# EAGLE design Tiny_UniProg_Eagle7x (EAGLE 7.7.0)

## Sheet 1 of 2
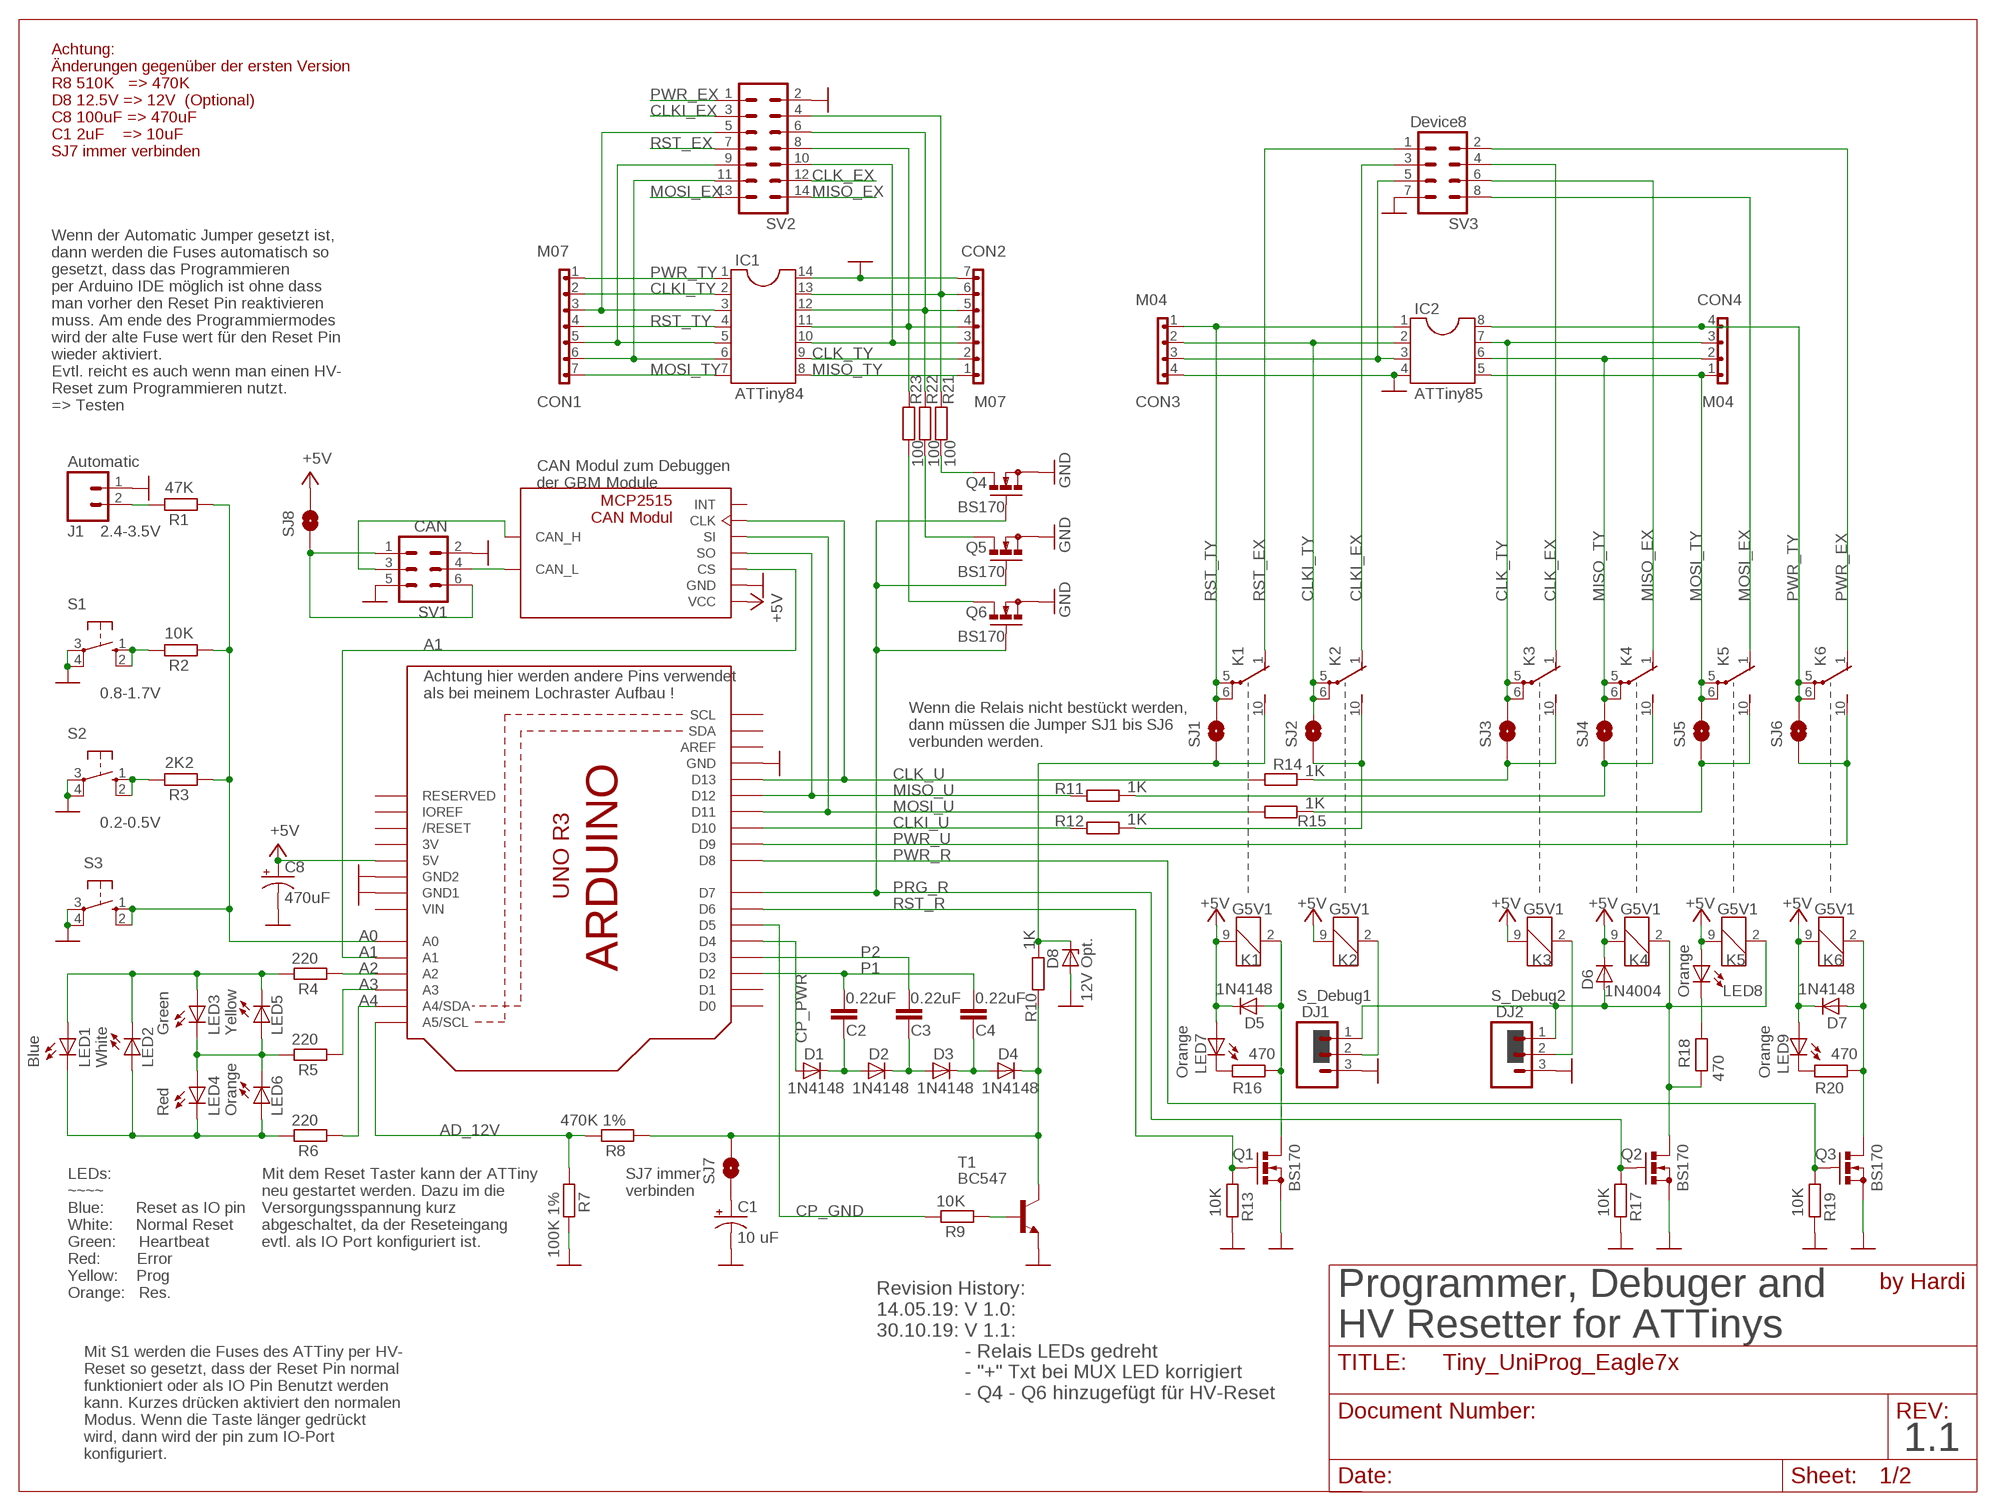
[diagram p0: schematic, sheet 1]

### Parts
C1  10 uF  100UF-25V-20%(PTH)D5MM  [CPOL-RADIAL-10UF-63V]
C2  0.22uF  C-EU050-024X044  [C050-024X044]
C3  0.22uF  C-EU050-024X044  [C050-024X044]
C4  0.22uF  C-EU050-024X044  [C050-024X044]
C8  470uF  SPARKFUN-CAPACITORS_100UF-25V-20%(PTH)  [SPARKFUN-CAPACITORS_CPOL-RADIAL-100UF-25V]
CAN1  MCP2515_CAN_MODUL  [MCP2515_CAN_MODUL]
CON1  M07  [1X07]
CON2  M07  [1X07]
CON3  M04  [1X04]
CON4  M04  [1X04]
D1  1N4148  1N4148DO35-2  [DO35-2]
D2  1N4148  1N4148DO35-2  [DO35-2]
D3  1N4148  1N4148DO35-2  [DO35-2]
D4  1N4148  1N4148DO35-2  [DO35-2]
D5  1N4148  1N4148DO35-2  [DO35-2]
D6  1N4004  1N4004DO35-2  [DO35-2]
D7  1N4148  1N4148DO35-2  [DO35-2]
D8  12V Opt.  ZENER-DIODEZD-2.5  [ZDIO-2.5]
DJ1  S_Debug1  M03PTH  [1X03]
DJ2  S_Debug2  M03PTH  [1X03]
IC1  ATTiny84  DIL14  [DIL14]
IC2  ATTiny85  DIL8  [DIL08]
J1  Automatic  M02PTH  [1X02]
K1  G5V1  [G5V1]
K2  G5V1  [G5V1]
K3  G5V1  [G5V1]
K4  G5V1  [G5V1]
K5  G5V1  [G5V1]
K6  G5V1  [G5V1]
LED1  Blue  LED3MM  [LED3MM]
LED2  White  LED3MM  [LED3MM]
LED3  Green  LED3MM  [LED3MM]
LED4  Red  LED3MM  [LED3MM]
LED5  Yellow  LED3MM  [LED3MM]
LED6  Orange  LED3MM  [LED3MM]
LED7  Orange  LED3MM  [LED3MM]
LED8  Orange  LED3MM  [LED3MM]
LED9  Orange  LED3MM  [LED3MM]
Q1  BS170  [SOT54E]
Q2  BS170  [SOT54E]
Q3  BS170  [SOT54E]
Q4  BS170  [SOT54E]
Q5  BS170  [SOT54E]
Q6  BS170  [SOT54E]
R1  47K  R0204/7  [0204/7]
R2  10K  R0204/7  [0204/7]
R3  2K2  R0204/2V  [0204/2V]
R4  220  R0204/2V  [0204/2V]
R5  220  R0204/2V  [0204/2V]
R6  220  R0204/2V  [0204/2V]
R7  100K 1%  R0204/2V  [0204/2V]
R8  470K 1%  R0204/7  [0204/7]
R9  10K  R0204/2V  [0204/2V]
R10  1K  R0204/2V  [0204/2V]
R11  1K  R0204/2V  [0204/2V]
R12  1K  R0204/2V  [0204/2V]
R13  10K  R0204/2V  [0204/2V]
R14  1K  R0204/2V  [0204/2V]
R15  1K  R0204/2V  [0204/2V]
R16  470  R0204/2V  [0204/2V]
R17  10K  R0204/2V  [0204/2V]
R18  470  R0204/2V  [0204/2V]
R19  10K  R0204/2V  [0204/2V]
R20  470  R0204/2V  [0204/2V]
R21  100  R0204/2V  [0204/2V]
R22  100  R0204/2V  [0204/2V]
R23  100  R0204/2V  [0204/2V]
S1  10-XX  [B3F-10XX]
S2  10-XX  [B3F-10XX]
S3  10-XX  [B3F-10XX]
SJ1  SOLDERJUMPERNO  [SJ_2S-NO]
SJ2  SOLDERJUMPERNO  [SJ_2S-NO]
SJ3  SOLDERJUMPERNO  [SJ_2S-NO]
SJ4  SOLDERJUMPERNO  [SJ_2S-NO]
SJ5  SOLDERJUMPERNO  [SJ_2S-NO]
SJ6  SOLDERJUMPERNO  [SJ_2S-NO]
SJ7  SOLDERJUMPERNO  [SJ_2S-NO]
SJ8  SOLDERJUMPERNO  [SJ_2S-NO]
SV1  CAN  ML6  [ML6]
SV2  ML14  [ML14]
SV3  Device8  CON-HARTING-ML_ML08  [CON-HARTING-ML_ML08]
T1  BC547  [TO92]
U1  ARDUINOR3-DIMENSION  [ARDUINOR3]

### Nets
+5V: C8.1(+) CAN1.1(VCC) D5.C D6.C D7.C K1.9 K2.9 K3.9 K4.9 K5.9 K6.9 LED7.A LED8.A LED9.A SJ8.2 U1.5V
A0: R1.1 R2.1 R3.1 S3.1(S) S3.2(S1) U1.A0
A1: CAN1.3(CS) U1.A1
A2: R4.1 U1.A2
A3: R5.1 U1.A3
A4: R6.1 U1.A4(A4/SDA)
AD_12V: R7.1 R8.2 U1.A5(A5/SCL)
CLK_EX: K3.1(2:O) SV2.12 SV3.4
CLK_TY: CON2.2 CON4.3 IC1.9 IC2.7 K3.5(2:P) K3.6(2:P) SJ3.2
CLK_U: CAN1.6(CLK) R14.1 U1.D13
CLKI_EX: K2.1(2:O) SV2.3 SV3.3
CLKI_TY: CON1.2 CON3.2 IC1.2 IC2.2 K2.5(2:P) K2.6(2:P) SJ2.2
CLKI_U: R12.1 U1.D10
CP_GND: R9.2 U1.D5
CP_PWR: D1.A U1.D4
GND: C1.2(-) C8.2(-) CAN1.2(GND) CON2.7 CON3.4 D8.A DJ1.3 DJ2.3 IC1.14 IC2.4 J1.1 Q1.S Q2.S Q3.S Q4.S Q5.S Q6.S R7.2 R13.2 R17.2 R19.2 S1.3(P) S1.4(P1) S2.3(P) S2.4(P1) S3.3(P) S3.4(P1) SV1.2 SV1.5 SV2.2 SV3.7 T1.1(E) U1.GND U1.GND1 U1.GND2
MISO_EX: K4.1(2:O) SV2.14 SV3.6
MISO_TY: CON2.1 CON4.2 IC1.8 IC2.6 K4.5(2:P) K4.6(2:P) SJ4.2
MISO_U: CAN1.4(SO) R11.1 U1.D12
MOSI_EX: K5.1(2:O) SV2.13 SV3.8
MOSI_TY: CON1.7 CON4.1 IC1.7 IC2.5 K5.5(2:P) K5.6(2:P) SJ5.2
MOSI_U: CAN1.5(SI) R15.1 U1.D11
N$1: C2.2 D1.C D2.A
N$2: C3.2 D2.C D3.A
N$3: C4.2 D3.C D4.A
N$6: CON2.3 IC1.10 SV2.10
N$7: R9.1 T1.2(B)
N$8: CAN1.8(CAN_L) SV1.4
N$9: D4.C R8.1 R10.2 SJ7.2 T1.3(C)
N$10: CAN1.9(CAN_H) SV1.3
N$11: CON2.4 IC1.11 R23.2 SV2.8
N$12: CON2.5 IC1.12 R22.2 SV2.6
N$13: K5.10(2:S) R15.2 SJ5.1
N$14: CON2.6 IC1.13 R21.2 SV2.4
N$15: K4.10(2:S) R11.2 SJ4.1
N$17: K3.10(2:S) R14.2 SJ3.1
N$19: DJ1.2 K2.2
N$20: D5.A K1.2 Q1.D R16.2
N$21: DJ2.2 K3.2
N$22: D8.C K1.10(2:S) R10.1 SJ1.1
N$23: CON1.6 IC1.6 SV2.11
N$24: K2.10(2:S) R12.2 SJ2.1
N$25: D7.A K6.2 Q3.D R20.2
N$26: D6.A DJ1.1 DJ2.1 K4.2 K5.2 Q2.D R18.2
N$27: CON1.5 IC1.5 SV2.9
N$28: J1.2 R1.2
N$30: CON1.3 IC1.3 SV2.5
N$33: R3.2 S2.1(S) S2.2(S1)
N$34: LED1.A LED2.K(C) LED3.A LED5.K(C) R4.2
N$36: LED7.K(C) R16.1
N$37: LED8.K(C) R18.1
N$38: LED9.K(C) R20.1
N$39: C1.1(+) SJ7.1
N$42: LED3.K(C) LED4.A LED5.A LED6.K(C) R5.2
N$44: LED1.K(C) LED2.A LED4.K(C) LED6.A R6.2
N$45: SJ8.1 SV1.1 SV1.6
N$48: CON3.3 IC2.3 SV3.5
N$67: R2.2 S1.1(S) S1.2(S1)
N$108: Q4.D R21.1
N$109: Q5.D R22.1
N$110: Q6.D R23.1
P1: C2.1 C4.1 U1.D2
P2: C3.1 U1.D3
PRG_R: Q2.G Q4.G Q5.G Q6.G R17.1 U1.D7
PWR_EX: K6.1(2:O) SV2.1 SV3.2
PWR_R: Q3.G R19.1 U1.D8
PWR_TY: CON1.1 CON4.4 IC1.1 IC2.8 K6.5(2:P) K6.6(2:P) SJ6.2
PWR_U: K6.10(2:S) SJ6.1 U1.D9
RST_EX: K1.1(2:O) SV2.7 SV3.1
RST_R: Q1.G R13.1 U1.D6
RST_TY: CON1.4 CON3.1 IC1.4 IC2.1 K1.5(2:P) K1.6(2:P) SJ1.2
Unconnected: CAN1.7(INT) U1.AREF U1.D0 U1.D1 U1.IOREF U1.RESERVED U1.RESET(/RESET) U1.SCL U1.SDA

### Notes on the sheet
- Achtung:
  Änderungen gegenüber der ersten Version
  R8 510K   => 470K
  D8 12.5V => 12V  (Optional)
  C8 100uF => 470uF
  C1 2uF    => 10uF
  SJ7 immer verbinden
- Wenn der Automatic Jumper gesetzt ist,
  dann werden die Fuses automatisch so
  gesetzt, dass das Programmieren
  per Arduino IDE möglich ist ohne dass
  man vorher den Reset Pin reaktivieren
  muss. Am ende des Programmiermodes
  wird der alte Fuse wert für den Reset Pin
  wieder aktiviert.
  Evtl. reicht es auch wenn man einen HV-
  Reset zum Programmieren nutzt.
  => Testen
- CAN Modul zum Debuggen 
  der GBM Module
- 2.4-3.5V
- 0.8-1.7V
- Achtung hier werden andere Pins verwendet
  als bei meinem Lochraster Aufbau !
- Wenn die Relais nicht bestückt werden,
  dann müssen die Jumper SJ1 bis SJ6
  verbunden werden.
- 0.2-0.5V
- LEDs:
  ~~~~
  Blue:       Reset as IO pin
  White:     Normal Reset
  Green:     Heartbeat
  Red:        Error
  Yellow:    Prog
  Orange:   Res.
- Mit dem Reset Taster kann der ATTiny
  neu gestartet werden. Dazu im die
  Versorgungsspannung kurz
  abgeschaltet, da der Reseteingang
  evtl. als IO Port konfiguriert ist.
- SJ7 immer
  verbinden
- Revision History:
  14.05.19: V 1.0: 
  30.10.19: V 1.1: 
                  - Relais LEDs gedreht 
                  - "+" Txt bei MUX LED korrigiert
                  - Q4 - Q6 hinzugefügt für HV-Reset
- by Hardi
- Programmer, Debuger and 
  HV Resetter for ATTinys
- Mit S1 werden die Fuses des ATTiny per HV-
  Reset so gesetzt, dass der Reset Pin normal
  funktioniert oder als IO Pin Benutzt werden
  kann. Kurzes drücken aktiviert den normalen
  Modus. Wenn die Taste länger gedrückt
  wird, dann wird der pin zum IO-Port 
  konfiguriert.
- 1.1

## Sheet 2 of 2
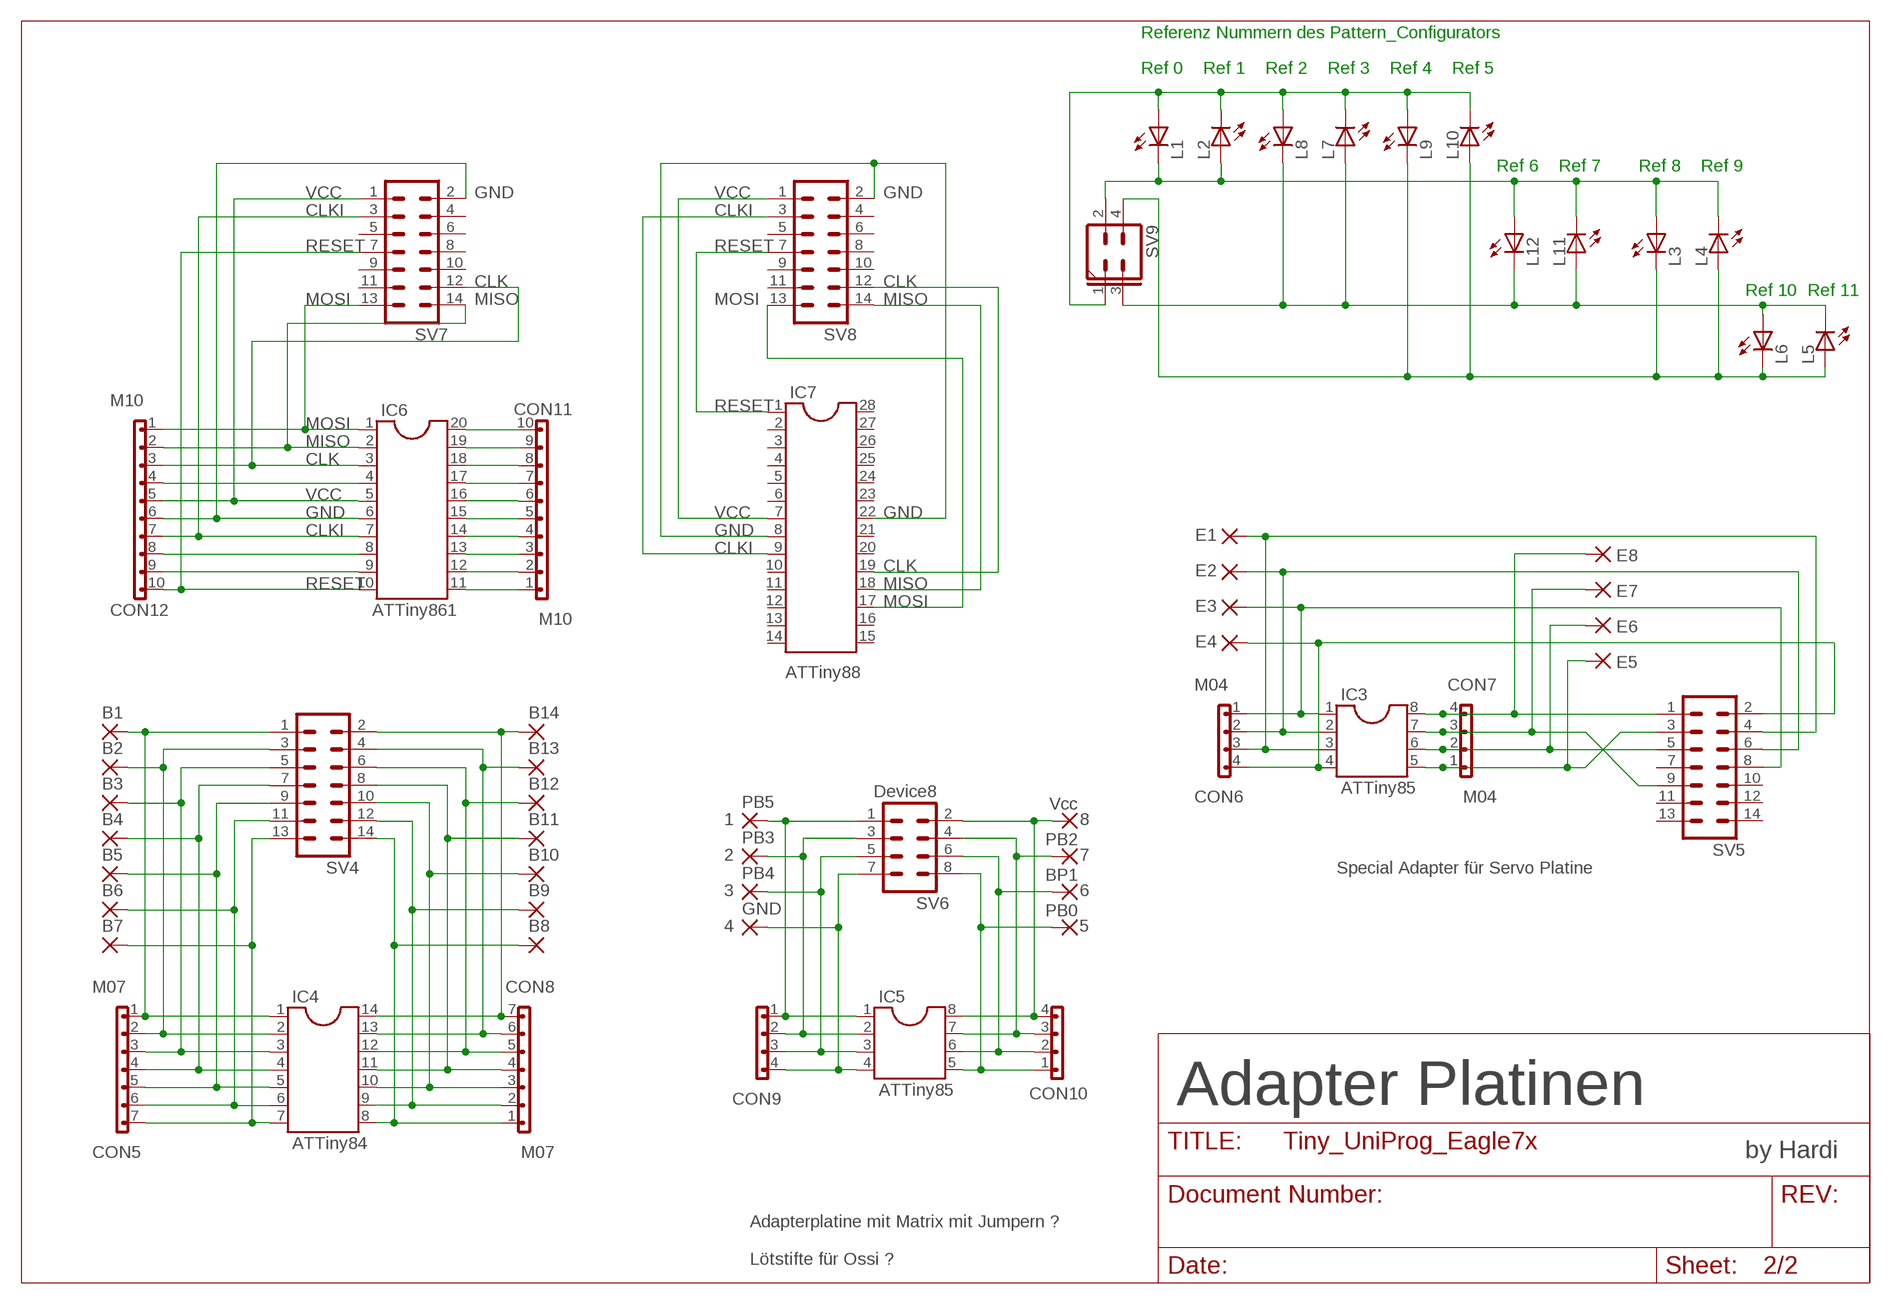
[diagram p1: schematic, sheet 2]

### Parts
1  PB5  2,54/1,0  [2,54/1,0]
2  PB3  2,54/1,0  [2,54/1,0]
3  PB4  2,54/1,0  [2,54/1,0]
4  GND  2,54/1,0  [2,54/1,0]
5  PB0  2,54/1,0  [2,54/1,0]
6  BP1  2,54/1,0  [2,54/1,0]
7  PB2  2,54/1,0  [2,54/1,0]
8  Vcc  2,54/1,0  [2,54/1,0]
B1  2,54/1,0  [2,54/1,0]
B2  2,54/1,0  [2,54/1,0]
B3  2,54/1,0  [2,54/1,0]
B4  2,54/1,0  [2,54/1,0]
B5  2,54/1,0  [2,54/1,0]
B6  2,54/1,0  [2,54/1,0]
B7  2,54/1,0  [2,54/1,0]
B8  2,54/1,0  [2,54/1,0]
B9  2,54/1,0  [2,54/1,0]
B10  2,54/1,0  [2,54/1,0]
B11  2,54/1,0  [2,54/1,0]
B12  2,54/1,0  [2,54/1,0]
B13  2,54/1,0  [2,54/1,0]
B14  2,54/1,0  [2,54/1,0]
CON5  M07  [1X07]
CON6  M04  [1X04]
CON7  M04  [1X04]
CON8  M07  [1X07]
CON9  M04  [1X04]
CON10  M04  [1X04]
CON11  M10  [1X10]
CON12  M10  [1X10]
E1  2,54/1,0  [2,54/1,0]
E2  2,54/1,0  [2,54/1,0]
E3  2,54/1,0  [2,54/1,0]
E4  2,54/1,0  [2,54/1,0]
E5  2,54/1,0  [2,54/1,0]
E6  2,54/1,0  [2,54/1,0]
E7  2,54/1,0  [2,54/1,0]
E8  2,54/1,0  [2,54/1,0]
IC3  ATTiny85  DIL8  [DIL08]
IC4  ATTiny84  DIL14  [DIL14]
IC5  ATTiny85  DIL8  [DIL08]
IC6  ATTiny861  DIL20  [DIL20]
IC7  DIL28-3  [DIL28-3]
L1  LED3MM  [LED3MM]
L2  LED3MM  [LED3MM]
L3  LED3MM  [LED3MM]
L4  LED3MM  [LED3MM]
L5  LED3MM  [LED3MM]
L6  LED3MM  [LED3MM]
L7  LED3MM  [LED3MM]
L8  LED3MM  [LED3MM]
L9  LED3MM  [LED3MM]
L10  LED3MM  [LED3MM]
L11  LED3MM  [LED3MM]
L12  LED3MM  [LED3MM]
SV4  ML14  [ML14]
SV5  ML14  [ML14]
SV6  Device8  CON-HARTING-ML_ML08  [CON-HARTING-ML_ML08]
SV7  ML14  [ML14]
SV8  ML14  [ML14]
SV9  MA02-2MUX-SIGNAL  [MUX-SIGNAL]

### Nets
N$4: 4.1(P) CON9.4 IC5.4 SV6.7
N$5: 3.1(P) CON9.3 IC5.3 SV6.5
N$16: 2.1(P) CON9.2 IC5.2 SV6.3
N$18: 1.1(P) CON9.1 IC5.1 SV6.1
N$29: 5.1(P) CON10.1 IC5.5 SV6.8
N$31: 6.1(P) CON10.2 IC5.6 SV6.6
N$32: 7.1(P) CON10.3 IC5.7 SV6.4
N$35: B8.1(P) CON8.1 IC4.8 SV4.14
N$40: B9.1(P) CON8.2 IC4.9 SV4.12
N$41: B10.1(P) CON8.3 IC4.10 SV4.10
N$43: B11.1(P) CON8.4 IC4.11 SV4.8
N$46: B12.1(P) CON8.5 IC4.12 SV4.6
N$47: B13.1(P) CON8.6 IC4.13 SV4.4
N$49: B14.1(P) CON8.7 IC4.14 SV4.2
N$50: B7.1(P) CON5.7 IC4.7 SV4.13
N$51: B6.1(P) CON5.6 IC4.6 SV4.11
N$52: B5.1(P) CON5.5 IC4.5 SV4.9
N$53: B4.1(P) CON5.4 IC4.4 SV4.7
N$54: B3.1(P) CON5.3 IC4.3 SV4.5
N$55: B2.1(P) CON5.2 IC4.2 SV4.3
N$56: B1.1(P) CON5.1 IC4.1 SV4.1
N$57: 8.1(P) CON10.4 IC5.8 SV6.2
N$58: CON7.4 E8.1(P) IC3.8 SV5.1
N$59: CON6.4 E4.1(P) IC3.4 SV5.2
N$60: CON7.3 E7.1(P) IC3.7 SV5.9
N$61: CON7.2 E6.1(P) IC3.6 SV5.5
N$62: CON7.1 E5.1(P) IC3.5 SV5.3
N$63: CON6.1 E3.1(P) IC3.1 SV5.8
N$64: CON6.2 E2.1(P) IC3.2 SV5.6
N$65: CON6.3 E1.1(P) IC3.3 SV5.4
N$66: CON12.10 IC6.10 SV7.7
N$68: CON12.7 IC6.7 SV7.3
N$69: CON12.6 IC6.6 SV7.2
N$70: CON12.5 IC6.5 SV7.1
N$71: CON12.3 IC6.3 SV7.12
N$72: CON12.2 IC6.2 SV7.14
N$73: CON12.1 IC6.1 SV7.13
N$74: CON12.4 IC6.4
N$75: CON12.8 IC6.8
N$76: CON12.9 IC6.9
N$77: CON11.1 IC6.11
N$78: CON11.2 IC6.12
N$79: CON11.3 IC6.13
N$80: CON11.4 IC6.14
N$81: CON11.5 IC6.15
N$82: CON11.6 IC6.16
N$83: CON11.7 IC6.17
N$84: CON11.8 IC6.18
N$85: CON11.9 IC6.19
N$86: CON11.10 IC6.20
N$87: IC7.9 SV8.3
N$88: IC7.8 IC7.22 SV8.2
N$89: IC7.7 SV8.1
N$90: IC7.1 SV8.7
N$91: IC7.17 SV8.13
N$92: IC7.18 SV8.14
N$93: L1.K(C) L2.A L3.A L4.K(C) L11.K(C) L12.A SV9.2
N$94: IC7.19 SV8.12
N$95: L1.A L2.K(C) L7.K(C) L8.A L9.A L10.K(C) SV9.1
N$97: L3.K(C) L4.A L5.A L6.K(C) L9.K(C) L10.A SV9.4
N$98: L5.K(C) L6.A L7.A L8.K(C) L11.A L12.K(C) SV9.3
Unconnected: IC7.2 IC7.3 IC7.4 IC7.5 IC7.6 IC7.10 IC7.11 IC7.12 IC7.13 IC7.14 IC7.15 IC7.16 IC7.20 IC7.21 IC7.23 IC7.24 IC7.25 IC7.26 IC7.27 IC7.28 SV5.7 SV5.10 SV5.11 SV5.12 SV5.13 SV5.14 SV7.4 SV7.5 SV7.6 SV7.8 SV7.9 SV7.10 SV7.11 SV8.4 SV8.5 SV8.6 SV8.8 SV8.9 SV8.10 SV8.11

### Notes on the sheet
- Referenz Nummern des Pattern_Configurators
- Ref 0 | Ref 1 | Ref 2 | Ref 3 | Ref 4 | Ref 5
- Ref 6 | Ref 7 | Ref 8 | Ref 9
- VCC | GND | VCC | GND
- CLKI | CLKI
- RESET | RESET
- CLK | CLK
- Ref 10 | Ref 11
- MOSI | MISO | MOSI | MISO
- RESET
- MOSI
- MISO
- CLK
- VCC
- GND | VCC | GND
- CLKI | GND
- CLKI
- CLK
- RESET | MISO
- MOSI
- ATTiny88
- Special Adapter für Servo Platine
- Adapter Platinen
- by Hardi
- Adapterplatine mit Matrix mit Jumpern ?
  
  Lötstifte für Ossi ?

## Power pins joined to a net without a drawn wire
3V: U1.3V
VIN: U1.VIN

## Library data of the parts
1-8 B1-B14 E1-E8 = wirepad:2,54/1,0: THROUGH-HOLE PAD
C1 = SparkFun-Capacitors:100UF-25V-20%(PTH): CAP-08439
C2-C4 = rcl:C-EU: CAPACITOR, European symbol; SPICEPREFIX: C
C8 = Sound_MP3-TF-16P_and_WS2811:SPARKFUN-CAPACITORS_100UF-25V-20%(PTH): CAP-08439; PROD_ID: CAP-08439
CAN1 = Arduino_fuer_LEDs_DCC_2_All:MCP2515_CAN_MODUL: MCP2515 CAN Modul
CON1 CON2 CON5 CON8 = Connectors_Inline3_7:M07
CON3 CON4 CON6 CON7 CON9 CON10 = Connectors_Inline3_7:M04
CON11 CON12 = Connectors_Inline3_7:M10
D1-D5 D7 = diode:1N4148: DIODE
D6 = diode:1N4004: DIODE
D8 = diode@1:ZENER-DIODE: Z-Diode
DJ1 DJ2 = SparkFun-Connectors:M03: Header 3 Standard 3-pin 0.1" header. Use with straight break away headers (SKU : PRT-00116), right angle break away headers (PRT-00553), swiss pins (PRT-00743), machine pins (PRT-00117), and female headers (PRT-00115). Molex polarized connector foot print use with SKU : PRT-08232 with associated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
IC1 IC4 = ic-package:DIL14: Dual In Line / Socket
IC2 IC3 IC5 = ic-package:DIL8: Dual In Line / Socket
IC6 = ic-package@1:DIL20: Dual In Line / Socket
IC7 = ic-package@1:DIL28: Dual In Line
J1 = SparkFun-Connectors:M02: Standard 2-pin 0.1" header. Use with
K1-K6 = relay:G5V1: RELAY 1 x switch, 0.5 A/125 V AC, 1 A/24 V DC , Omron; MPN: G5V-1-DC24; OC_FARNELL: 9949593; OC_NEWARK: 36M6377
L1-L12 LED1-LED9 = Arduino_fuer_LEDs_DCC_2:LED: LED
Q1-Q6 = transistor-small-signal:BS170: N-CHANNEL MOS FET
R1 R2 R8 = Arduino_fuer_LEDs_DCC_2:R: RESISTOR, European symbol; SPICEMODEL: NONE; SPICEPREFIX: R
R3-R7 R9-R23 = Arduino_fuer_LEDs_DCC_2:R: RESISTOR, European symbol
S1-S3 = switch-omron:10-XX: OMRON SWITCH; MPN: B3F-1000; OC_FARNELL: 176432; OC_NEWARK: 36M3542
SJ1-SJ8 = SparkFun-Retired:SOLDERJUMPER: Solder Jumper
SV1 = Arduino_fuer_LEDs_DCC_2:ML6: HARTING; OC_FARNELL: unknown; OC_NEWARK: unknown
SV2 SV4 SV5 SV7 SV8 = Arduino_fuer_LEDs_DCC_2:ML14: HARTING; OC_FARNELL: unknown; OC_NEWARK: unknown
SV3 SV6 = PushButtonAction_4017_2:CON-HARTING-ML_ML08: Modified by Hardi; OC_FARNELL: unknown; OC_NEWARK: unknown
SV9 = con-lstb:MA02-2: PIN HEADER
T1 = transistor:BC547: NPN TRANSISTOR
U1 = adafruit:ARDUINOR3: This is a new object for the new Arduino R3 - with extra pins that you may want to use (such as IOref, and duplicated A4/A5

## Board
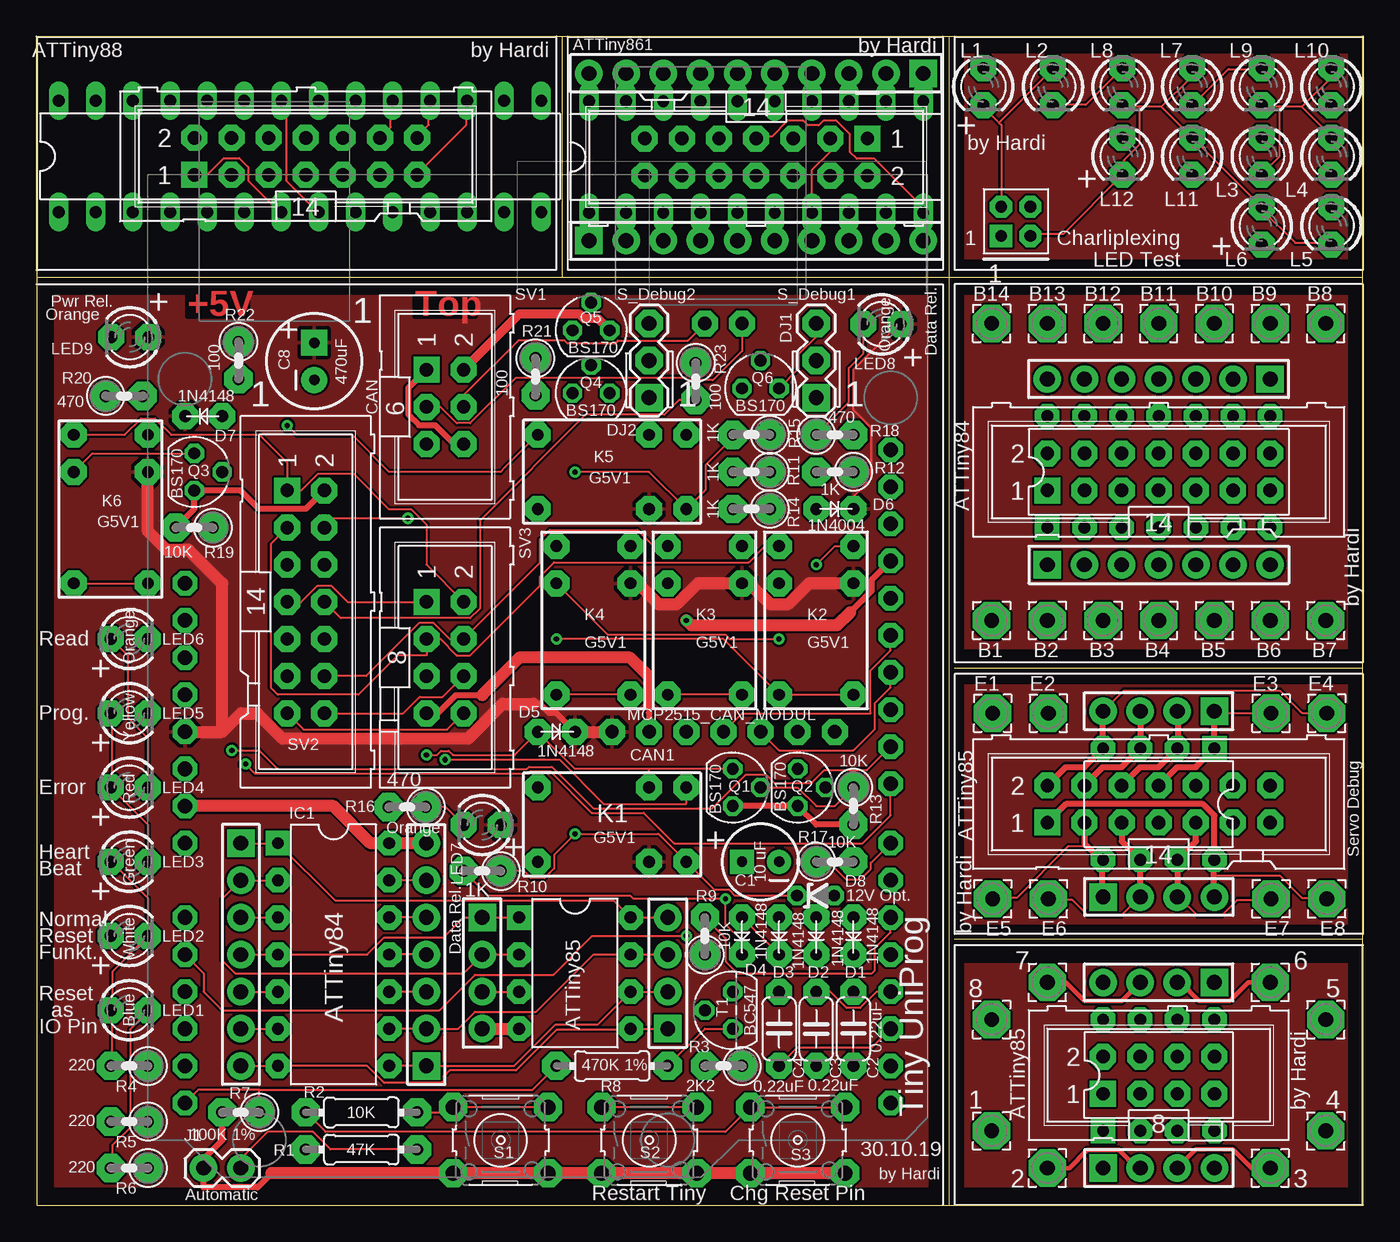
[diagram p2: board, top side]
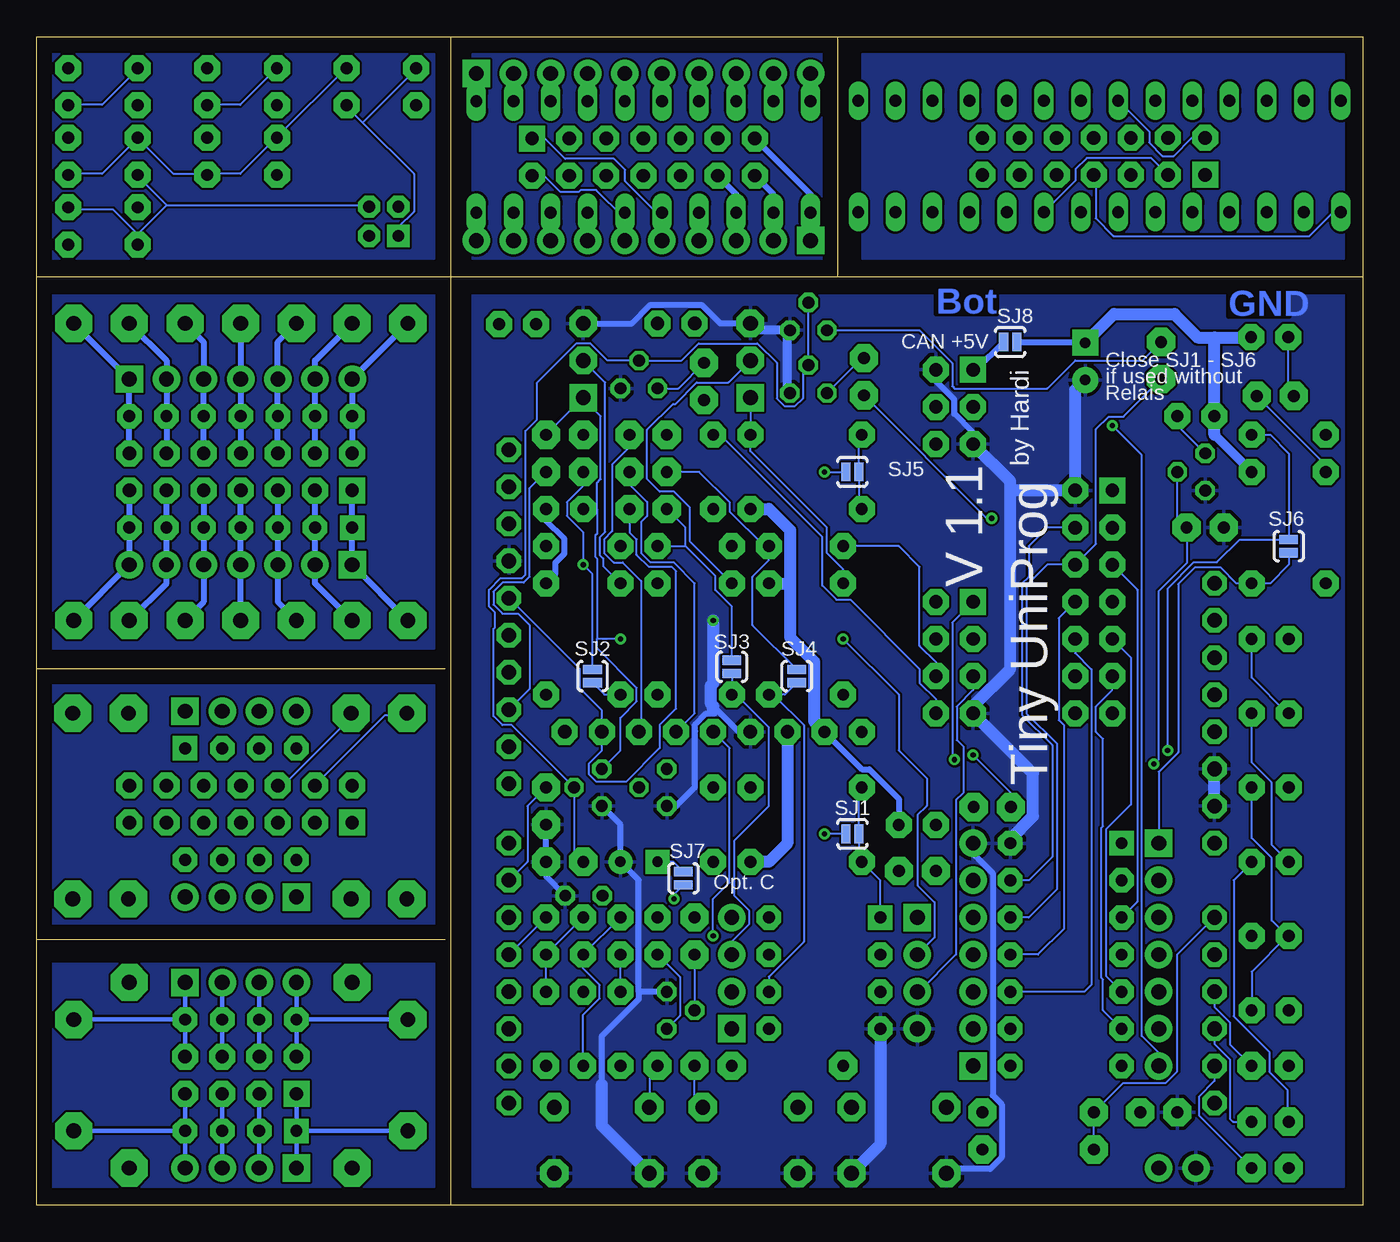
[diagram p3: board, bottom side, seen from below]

Size 90.74 x 79.95 mm. Coordinates in mm from the lower left corner, seen from the top.
Outline: 62.4,0 90.74,0 90.74,36.73
Outline: 90.74,36.73 90.74,63.5
Outline: 90.74,63.5 90.74,79.95 62.4,79.95
Outline: 0,63.5 0,79.95 62.4,79.95
Outline: 0,63.5 0,0 62.4,0
Outline: 0,63.5 35.96,63.5
Outline: 35.96,63.5 90.74,63.5
Outline: 62.4,79.95 62.4,0
Outline: 90.74,18.18 62.8,18.18
Outline: 90.74,36.73 62.8,36.73
Outline: 35.96,79.9 35.96,63.5
Copper layers (1*16): Top 0.035mm / dielectric 1.5mm / Bottom 0.035mm
Design rules "default": minimum track width 6mil, minimum drill 0.35mm, track to track 6mil, track to pad 6mil, pad to pad 6mil, via to via 6mil, smd to smd 6mil, copper to edge 40mil, drill to drill 6mil, minimum pad ring 10mil, minimum via ring 8mil, stop-mask expansion 4mil, vias tented up to drill 0mil, thermal gap 10mil

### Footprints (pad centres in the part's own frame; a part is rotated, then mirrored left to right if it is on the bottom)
2,54/1,0 = drill 1.016 pad 2.54 octagon: 1 0,0
CPOL-RADIAL-10UF-63V = drill 0.7 pad 1.651 square: 1 1.27,0 | drill 0.7 pad 1.651: 2 -1.27,0
C050-024X044 = drill 0.813 pad 1.778 octagon: 1 -2.54,0; 2 2.54,0
SPARKFUN-CAPACITORS_CPOL-RADIAL-100UF-25V = drill 0.7 pad 1.778 square: 1 1.27,0 | drill 0.7 pad 1.778: 2 -1.27,0
MCP2515_CAN_MODUL = drill 0.914 pad 1.778 octagon: 1 0,0; 2 0,-2.54; 3 0,-5.08; 4 0,-7.62; 5 0,-10.16; 6 0,-12.7; 7 0,-15.24; 8 27.94,-6.35; 9 27.94,-8.89
1X07 = drill 1.016 pad 1.88 square: 1 0,0 | drill 1.016 pad 1.88: 2 2.54,0; 3 5.08,0; 4 7.62,0; 5 10.16,0; 6 12.7,0; 7 15.24,0
1X04 = drill 1.016 pad 1.88 square: 1 0,0 | drill 1.016 pad 1.88: 2 2.54,0; 3 5.08,0; 4 7.62,0
1X10 = drill 1.016 pad 1.88 square: 1 0,0 | drill 1.016 pad 1.88: 2 2.54,0; 3 5.08,0; 4 7.62,0; 5 10.16,0; 6 12.7,0; 7 15.24,0; 8 17.78,0; 9 20.32,0; 10 22.86,0
DO35-2 = drill 0.813 pad 1.778 octagon: A 1.27,0; C -1.27,0
ZDIO-2.5 = drill 0.813 octagon: A 1.27,0; C -1.27,0
1X03 = drill 1.016 pad 1.88 square: 1 0,0 | drill 1.016 pad 1.88 octagon: 2 2.54,0; 3 5.08,0
DIL14 = drill 0.813 pad 1.676 square: 1 -7.62,-3.81 | drill 0.813 pad 1.676 octagon: 2 -5.08,-3.81; 3 -2.54,-3.81; 4 0,-3.81; 5 2.54,-3.81; 6 5.08,-3.81; 7 7.62,-3.81; 8 7.62,3.81; 9 5.08,3.81; 10 2.54,3.81; 11 0,3.81; 12 -2.54,3.81; 13 -5.08,3.81; 14 -7.62,3.81
DIL08 = drill 0.813 pad 1.676 square: 1 -3.81,-3.81 | drill 0.813 pad 1.676 octagon: 2 -1.27,-3.81; 3 1.27,-3.81; 4 3.81,-3.81; 5 3.81,3.81; 6 1.27,3.81; 7 -1.27,3.81; 8 -3.81,3.81
DIL20 = drill 0.813 long: 1 -11.43,-3.81; 2 -8.89,-3.81; 3 -6.35,-3.81; 4 -3.81,-3.81; 5 -1.27,-3.81; 6 1.27,-3.81; 7 3.81,-3.81; 8 6.35,-3.81; 9 8.89,-3.81; 10 11.43,-3.81; 11 11.43,3.81; 12 8.89,3.81; 13 6.35,3.81; 14 3.81,3.81; 15 1.27,3.81; 16 -1.27,3.81; 17 -3.81,3.81; 18 -6.35,3.81; 19 -8.89,3.81; 20 -11.43,3.81
DIL28-3 = drill 0.813 long: 1 -16.51,-3.81; 2 -13.97,-3.81; 3 -11.43,-3.81; 4 -8.89,-3.81; 5 -6.35,-3.81; 6 -3.81,-3.81; 7 -1.27,-3.81; 8 1.27,-3.81; 9 3.81,-3.81; 10 6.35,-3.81; 11 8.89,-3.81; 12 11.43,-3.81; 13 13.97,-3.81; 14 16.51,-3.81; 15 16.51,3.81; 16 13.97,3.81; 17 11.43,3.81; 18 8.89,3.81; 19 6.35,3.81; 20 3.81,3.81; 21 1.27,3.81; 22 -1.27,3.81; 23 -3.81,3.81; 24 -6.35,3.81; 25 -8.89,3.81; 26 -11.43,3.81; 27 -13.97,3.81; 28 -16.51,3.81
1X02 = drill 1.016 pad 1.88: 1 0,0; 2 2.54,0
G5V1 = drill 0.813 pad 1.778 octagon: 1 -5.08,-2.54; 2 -2.54,-2.54; 5 5.08,-2.54; 6 5.08,2.54; 9 -2.54,2.54; 10 -5.08,2.54
LED3MM = drill 0.813 pad 1.778 octagon: A -1.27,0; K 1.27,0
SOT54E = drill 0.813 octagon: D -1.27,0; G 0,1.905; S 1.27,0
0204/7 = drill 0.813 pad 1.93 octagon: 1 -3.81,0; 2 3.81,0
0204/2V = drill 0.813 pad 1.93 octagon: 1 -1.27,0; 2 1.27,0
B3F-10XX = drill 1.016 pad 1.93 octagon: 1 -3.251,2.261; 2 3.251,2.261; 3 -3.251,-2.261; 4 3.251,-2.261
SJ_2S-NO = smd 0.635 x 1.27: 1 -0.45,0; 2 0.45,0
ML6 = drill 0.914 pad 1.778 square: 1 -2.54,-1.27 | drill 0.914 pad 1.778 octagon: 2 -2.54,1.27; 3 0,-1.27; 4 0,1.27; 5 2.54,-1.27; 6 2.54,1.27
ML14 = drill 0.914 pad 1.778 square: 1 -7.62,-1.27 | drill 0.914 pad 1.778 octagon: 2 -7.62,1.27; 3 -5.08,-1.27; 4 -5.08,1.27; 5 -2.54,-1.27; 6 -2.54,1.27; 7 0,-1.27; 8 0,1.27; 9 2.54,-1.27; 10 2.54,1.27; 11 5.08,-1.27; 12 5.08,1.27; 13 7.62,-1.27; 14 7.62,1.27
CON-HARTING-ML_ML08 = drill 0.914 pad 1.778 square: 1 -5.08,-1.27 | drill 0.914 pad 1.778 octagon: 2 -5.08,1.27; 3 -2.54,-1.27; 4 -2.54,1.27; 5 0,-1.27; 6 0,1.27; 7 2.54,-1.27; 8 2.54,1.27
MUX-SIGNAL = drill 0.8 pad 1.524 square: 1 -1,-1 | drill 0.8 pad 1.524 octagon: 2 -1,1; 3 1,-1; 4 1,1
TO92 = drill 0.813 octagon: 1 1.27,0; 2 0,1.905; 3 -1.27,0
ARDUINOR3 = drill 1 pad 1.676 octagon: 3V 35.56,2.54; 5V 38.1,2.54; A0 50.8,2.54; A1 53.34,2.54; A2 55.88,2.54; A3 58.42,2.54; A4 60.96,2.54; A5 63.5,2.54; AREF 23.876,50.8; D0 63.5,50.8; D1 60.96,50.8; D2 58.42,50.8; D3 55.88,50.8; D4 53.34,50.8; D5 50.8,50.8; D6 48.26,50.8; D7 45.72,50.8; D8 41.656,50.8; D9 39.116,50.8; D10 36.576,50.8; D11 34.036,50.8; D12 31.496,50.8; D13 28.956,50.8; GND 26.416,50.8; GND1 43.18,2.54; GND2 40.64,2.54; IOREF 30.48,2.54; RESERVED 27.94,2.54; RESET 33.02,2.54; SCL 18.796,50.8; SDA 21.336,50.8; VIN 45.72,2.54

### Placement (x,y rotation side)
1  65.34,5.08 0 top
2  69.15,2.54 0 top
3  84.39,2.54 0 top
4  88.2,5.08 0 top
5  88.2,12.7 0 top
6  84.39,15.24 0 top
7  69.15,15.24 0 top
8  65.34,12.7 0 top
B1  65.34,40.01 0 top
B2  69.15,40.01 0 top
B3  72.96,40.01 0 top
B4  76.77,40.01 0 top
B5  80.58,40.01 0 top
B6  84.39,40.01 0 top
B7  88.2,40.01 0 top
B8  88.2,60.33 0 top
B9  84.39,60.33 0 top
B10  80.58,60.33 0 top
B11  76.77,60.33 0 top
B12  72.96,60.33 0 top
B13  69.15,60.33 0 top
B14  65.34,60.33 0 top
C1  49.53,23.5 180 top
C2  55.88,12.06 90 top
C3  53.34,12.06 270 top
C4  50.8,12.06 90 top
C8  19,57.73 90 top
CAN1  39.37,32.38 90 top
CON1  13.97,24.77 270 top
CON2  26.67,9.53 90 top
CON3  30.48,19.68 270 top
CON4  43.18,12.06 90 top
CON5  69.15,43.81 0 top
CON6  80.58,33.79 180 top
CON7  72.96,21.09 0 top
CON8  84.39,56.52 180 top
CON9  72.96,2.54 0 top
CON10  80.58,15.24 180 top
CON11  60.66,77.42 180 top
CON12  37.8,65.99 0 top
D1  55.88,18.41 90 top
D2  53.34,18.41 90 top
D3  50.8,18.41 90 top
D4  48.26,18.41 90 top
D5  35.56,32.38 180 top
D6  54.61,47.62 180 top
D7  11.43,53.98 0 top
D8  53.3,21.18 0 top
DJ1  53.34,55.24 90 top
DJ2  41.91,55.24 90 top
E1  65.41,33.66 0 top
E2  69.22,33.66 0 top
E3  84.45,33.66 0 top
E4  88.27,33.66 0 top
E5  65.41,20.95 180 top
E6  69.22,20.95 180 top
E7  84.45,20.95 180 top
E8  88.27,20.95 180 top
IC1  20.32,17.14 270 top
IC2  36.83,15.88 270 top
IC3  76.77,27.44 180 top
IC4  76.77,50.16 0 top
IC5  76.77,8.89 0 top
IC6  49.23,71.7 0 top
IC7  18.02,71.75 0 top
J1  11.43,2.54 0 top
K1  39.37,26.04 180 top
K2  53.34,40.01 270 top
K3  45.72,40.01 270 top
K4  38.1,40.01 270 top
K5  39.37,50.16 180 top
K6  5.08,47.62 270 top
L1  64.77,76.52 270 top
L2  69.53,76.52 270 top
L3  83.82,71.75 270 top
L4  88.58,71.75 270 top
L5  88.58,66.99 270 top
L6  83.82,66.99 270 top
L7  79.06,76.52 270 top
L8  74.3,76.52 270 top
L9  83.82,76.52 270 top
L10  88.58,76.52 270 top
L11  79.06,71.75 270 top
L12  74.3,71.75 270 top
LED1  6.35,13.34 0 top
LED2  6.35,18.41 0 top
LED3  6.35,23.5 0 top
LED4  6.35,28.57 0 top
LED5  6.35,33.66 0 top
LED6  6.35,38.73 0 top
LED7  30.49,26.01 180 top
LED8  57.83,60.27 180 top
LED9  6.38,59.38 180 top
Q1  47.62,28.57 270 top
Q2  52.07,28.57 270 top
Q3  10.79,50.16 270 top
Q4  37.94,55.56 0 top
Q5  37.94,59.85 0 top
Q6  49.53,55.88 0 top
R1  22.23,3.81 0 top
R2  22.23,6.35 0 top
R3  46.99,9.53 180 top
R4  6.35,9.53 180 top
R5  6.35,5.71 180 top
R6  6.35,2.54 180 top
R7  13.97,6.35 180 top
R8  39.37,9.53 180 top
R9  45.72,18.41 90 top
R10  30.48,22.86 180 top
R11  48.9,50.16 180 top
R12  54.61,50.16 180 top
R13  55.88,27.3 270 top
R14  48.9,47.62 180 top
R15  48.9,52.7 180 top
R16  25.36,27.23 180 top
R17  54.61,23.5 0 top
R18  54.61,52.7 0 top
R19  10.79,46.35 180 top
R20  6,55.37 0 top
R21  34.13,56.67 270 top
R22  13.81,57.78 270 top
R23  45.09,56.36 270 top
S1  31.75,4.45 0 top
S2  41.91,4.45 0 top
S3  52.07,4.45 0 top
SJ1  34.92,25.4 0 bottom
SJ2  52.7,36.2 270 bottom
SJ3  43.18,36.83 270 bottom
SJ4  38.73,36.2 270 bottom
SJ5  34.92,50.16 0 bottom
SJ6  5.08,45.09 270 bottom
SJ7  46.48,22.36 270 bottom
SJ8  24.13,59.05 0 bottom
SV1  27.94,54.61 270 top
SV2  18.41,41.27 270 top
SV3  27.94,36.2 270 top
SV4  76.77,50.16 0 top
SV5  76.77,27.44 0 top
SV6  78.04,8.89 0 top
SV7  49.23,71.7 180 top
SV8  18.41,71.75 0 top
SV9  66.99,67.31 0 top
T1  47.62,13.34 90 top
U1  7.62,70.48 270 top

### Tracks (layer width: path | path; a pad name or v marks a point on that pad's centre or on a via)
+5V
  Top 0.152: D6.C 55.88,48.48 57.07,49.67 57.07,53.2 55.88,54.39 55.88,57.15 58.99,60.27 LED8.A
  Top 0.406: 33.97,34.29 34.44,34.29 35.04,33.68 35.53,33.68 D5.C
  Top 0.813: D5.C CAN1.1 | U1.5V 12.7,32.38 | 12.7,32.38 13.97,33.66 15.1,33.66 16.85,31.9 29.5,31.9 31.89,34.29 33.97,34.29 | 12.7,32.38 12.7,42.55 10.41,44.83 8.89,44.83 7.62,46.1 K6.9 | K2.9 52.85,42.55 51.4,41.1 50.2,41.1 48.75,42.55 K3.9 45.23,42.55 43.78,41.1 42.58,41.1 41.13,42.55 K4.9
  Bottom 0.406: K2.9 55.24,43.18 55.24,43.96 54.63,44.57 54.63,45.6 55.88,46.84 D6.C | D5.C 34.27,29.82 33.77,29.82 31.76,27.8 LED7.A | SJ8.2 19.05,59.05 C8.1
  Bottom 0.61: K6.9 10.16,52.7
  Bottom 0.813: CAN1.1 39.37,24.77 40.64,23.5 K1.9 | K5.9 40.64,47.62 39.19,46.18 39.19,42.55 | 10.16,52.7 D7.C 10.16,59.37 | D5.C 37.54,33.1 37.54,37.19 39.19,38.84 39.19,42.55 | K4.9 39.19,42.55 | 10.16,59.37 7.67,59.37 LED9.A | C8.1 17.04,60.96 12.9,60.96 11.3,59.37 10.16,59.37
  pour Top: 1.27,62.23 60.96,62.23 60.96,1.27 1.27,1.27
A0
  Top 0.152: S3.2 S3.1 47.12,5 19.76,5 R2.1
  Bottom 0.152: R3.1 48.82,8.97 S3.1 | U1.A0 12.7,17.14 12.7,9.14 13.49,8.36 16.41,8.36 R2.1 R1.1
A1  (via drill 0.35)
  Top 0.152: U1.A1 11.43,15.88 11.43,14.61 12.7,13.34 27.56,13.34 30,15.77 35.36,15.77 38,18.41 v44.45,18.41
  Bottom 0.152: v44.45,18.41 44.45,20.95 43.33,22.07 43.33,31.27 CAN1.3
A2
  Bottom 0.152: U1.A2 10.16,13.57 9.09,12.51 9.09,11 R4.1
A3
  Bottom 0.152: U1.A3 10.16,11.03 9.09,9.97 9.09,5.92 8.89,5.71 R5.1
A4
  Bottom 0.152: U1.A4 10.16,8.49 11.23,7.43 11.23,6.15 R6.1
AD_12V
  Top 0.152: R8.2 33.93,7.9 15.24,7.9 | 15.24,7.9 11.07,7.9 U1.A5 | R7.1 15.24,7.9
CLK_EX
  Top 0.152: K3.1 42.22,45.09 41.1,46.2 35.1,46.2 34.44,45.55 34.44,43.97 SV3.4 28.25,38.73 27.13,39.85 26.21,39.85 22.55,36.2 SV2.12
CLK_TY
  Top 0.152: IC1.9 CON2.2 28.83,12.06 30,13.23 34.19,13.23 38.1,17.14 IC2.7 CON4.3 | K3.6 K3.5
  Bottom 0.152: CON4.3 43.18,18.03 42.01,19.2 42.01,20.17 43.03,21.18 43.03,24.92 40.64,27.3 40.64,32.7 42.72,34.77 43.03,34.77 K3.5 SJ3.2
CLK_U
  Bottom 0.152: U1.D13 53.57,36.68 53.57,35.33 52.07,33.83 CAN1.6 52.07,31.1 52.96,30.21 52.96,29.48 52.44,28.96 50.42,28.96 48.11,31.27 48.11,32.85 46.99,33.97 46.99,43.38 47.27,43.66 48.85,43.66 49.68,44.5 49.68,45.55 50.16,46.03 R14.1
CLKI_EX
  Top 0.152: SV2.3 16.03,45.24 16.03,35.41 16.51,34.92 22.02,34.92 24.71,37.62 26.67,37.62 SV3.3 27.63,38.73 28.75,37.62 29.67,37.62 34.44,42.39 34.44,43.01 35.4,43.97 48.72,43.97 49.84,45.09 K2.1
CLKI_TY  (via drill 0.35)
  Top 0.152: IC1.2 CON1.2 12.7,20.95 12.7,16.76 13.59,15.88 29.21,15.88 CON3.2 IC2.2 | K2.6 K2.5 46.99,38.73 v35.56,38.73
  Bottom 0.152: SJ2.2 51.88,34.92 K2.5 | v35.56,38.73 31.75,34.92 31.75,31.11 29.84,29.21 29.84,27.32 30.48,26.68 30.48,21.89 29.31,20.72 29.31,18.31 CON3.2
CLKI_U
  Bottom 0.152: U1.D10 57,35.33 57,39.68 57.78,40.46 58.86,40.46 59.49,41.09 59.49,41.97 58.86,42.6 57.41,42.6 57,43.01 57,49.05 R12.1
CP_GND
  Top 0.152: R9.2 47.14,18.26 47.14,16.68 47.95,15.88 57.15,15.88 57.35,16.08 57.35,17.59 58.42,18.65 U1.D5
CP_PWR
  Bottom 0.152: U1.D4 D1.A
GND  (via drill 0.35)
  Top 0.152: Q6.S 52.17,57.25 52.17,58.27 53.34,59.44 DJ1.3
  Top 0.406: S3.3 S2.4 S2.3 S1.4 S1.3 17.78,2.18 | 16.08,2.18 15.12,1.22 11.43,1.22 J1.1 11.43,3.17 12.7,4.45 R7.2 | 22.86,24.77 IC1.14 CON2.7 | R19.2 10.79,47.62 Q3.S 13.97,48.9 15.24,47.62 18.41,47.62 SV2.2 | R13.2 53.34,26.04 Q2.S Q1.S | SV3.7 27.45,33.66 28.69,34.9 30.48,34.9 | 41.88,36.17 41.88,33.68 41.91,33.66 CAN1.2 | U1.GND 57.12,42.77 57.12,42.03 55.65,40.55
  Top 0.61: Q5.S 38.42,60.64 37.46,60.64 37.13,60.97 36.21,60.97 36.2,60.96 33.02,60.96 SV1.2
  Top 0.813: v44.45,40.01 44.78,39.67 54.77,39.67 55.65,40.55 | S3.4 S3.3 17.78,2.18 16.08,2.18 | CON3.4 IC2.4 | 41.88,36.17 40.59,37.47 33.02,37.47 33.02,37.44 30.48,34.9 | CON2.7 22.86,24.77 20.32,27.3 U1.GND1
  Bottom 0.152: 55.88,22.48 R17.2
  Bottom 0.406: CON2.7 26.67,24.06 25.32,22.71 25.32,7.51 24.71,6.9 24.71,3.26 25.49,2.49 28.19,2.49 S1.3 | 52.07,8.26 52.07,11.57 49.55,14.09 49.55,14.61 | T1.1 49.55,14.61 | R17.2 R13.2 | Q2.S 50.8,26.04 C1.2 49.55,22.25 49.55,14.61 | SV1.5 26.67,52.85 27.96,54.15 27.96,55.13 29.21,56.37 SV1.2 | CAN1.2 42.69,32.38 42.69,32.39 44.45,34.15 | Q1.S 46.99,27.3 45.72,28.57 45.72,32.38 45.7,32.41 45.7,32.9 44.97,33.63 44.65,33.63 44.45,33.83 | D8.A 55.88,22.48 | DJ1.3 50.02,60.33 48.78,61.57 45.2,61.57 43.96,60.33 DJ2.3
  Bottom 0.61: Q5.S 39.37,59.85 | 39.37,59.85 41.43,59.85 DJ2.3 | Q4.S 39.37,55.72 39.37,59.85
  Bottom 0.813: 24.13,48.9 24.13,49.53 SV1.5 | 24.13,48.9 SV2.2 19.68,55.77 C8.2 | v44.45,40.01 44.45,35.7 44.63,35.52 44.63,34.33 44.45,34.15 44.45,33.83 | IC2.4 33.02,4.17 S1.4 | S3.3 52.07,5.44 52.07,8.26 | 24.13,48.9 24.13,36.69 26.67,34.15 SV3.7 22.57,29.55 22.57,26.6 24.13,25.04 IC1.14 | U1.GND1 U1.GND2
  pour Bottom: 1.27,62.23 60.96,62.23 60.96,1.27 1.27,1.27
MISO_EX
  Top 0.152: SV2.14 25.09,33.66 26.21,34.77 27.79,34.77 SV3.6
  Bottom 0.152: SV3.6 29.21,37.15 30.33,38.27 30.33,43.66 31.75,45.09 K4.1
MISO_TY
  Top 0.152: IC1.8 CON2.1 32.66,9.53 35.51,12.37 38.41,12.37 IC2.6 CON4.2 | K4.6 K4.5
  Bottom 0.152: SJ4.2 39.55,34.92 K4.6 40.49,34.77 40.18,34.77 38.25,32.85 38.25,18.02 40.64,15.64 IC2.6
MISO_U
  Top 0.152: CAN1.4 48.26,33.66 57.05,33.66 57.05,36.59 58.42,37.96 U1.D12
  Bottom 0.152: R11.1 50.16,49.31 48.97,48.12 48.97,47.13 49.38,46.72 49.38,44.62 48.72,43.97 47.14,43.97 45.72,42.55 45.72,33.66 CAN1.4
MOSI_EX
  Top 0.152: SV2.13 18.26,32.54 28.09,32.54 SV3.8
  Bottom 0.152: SV3.8 29.21,34.61 30.33,35.73 30.33,36.68 35.08,41.43 36.02,41.43 36.98,42.39 36.98,45.7 43.99,52.7 K5.1
MOSI_TY  (via drill 0.35)
  Top 0.152: CON1.7 IC1.7 22.62,9.53 23.79,8.36 27.7,8.36 27.84,8.49 27.84,8.79 28.27,9.22 32.79,9.22 35.6,12.03 40.6,12.03 IC2.5 CON4.1 | v17.14,53.34 17.78,52.7 21.59,52.7 24.13,50.16 31.75,50.16 32.07,50.48 K5.5
  Bottom 0.152: CON1.7 13.97,10.41 15.14,11.58 15.14,51.33 v17.14,53.34 | K5.6 34.48,47.81 SJ5.2 34.48,52.52 K5.5
MOSI_U
  Top 0.152: CAN1.5 50.8,31.11 55.88,31.11 57.35,32.59 57.35,34.35 58.42,35.42 U1.D11
  Bottom 0.152: R15.1 50.16,51.85 51.36,50.66 51.36,46.11 51.92,45.55 51.92,44.62 51.26,43.97 50.64,43.97 49.38,42.7 49.38,32.54 CAN1.5
N$1
  Bottom 0.152: C2.2 D1.C D2.A
N$2
  Bottom 0.152: C3.2 53.34,13.02 52.22,14.14 52.22,15.07 53.34,16.19 D2.C D3.A
N$3
  Top 0.152: D3.C D4.A
  Bottom 0.152: C4.2 D3.C
N$4
  Bottom 0.305: CON9.4 IC5.4 | IC5.4 SV6.7 | IC5.4 4.1
N$5
  Top 0.305: 3.1 83.12,2.54 81.85,3.81 79.31,3.81 CON9.3
  Bottom 0.305: SV6.5 IC5.3 CON9.3
N$6
  Top 0.152: CON2.3 IC1.10
  Bottom 0.152: SV2.10 19.68,37.78 18.57,36.66 18.57,15.09 19.05,14.61 IC1.10
N$7
  Bottom 0.152: R9.1 T1.2
N$8
  Top 0.152: CAN1.8 44.55,59.16 39.78,59.16 39.58,58.96 36.3,58.96 36.11,59.16 32.96,59.16 29.21,55.4 SV1.4
N$9  (via drill 0.35)
  Top 0.152: R8.1 45.72,12.06 T1.3 | D4.C 48.26,18.1 47.14,19.22 v47.14,20.95 40.84,20.95 40.64,21.16 30.91,21.16 R10.2
  Bottom 0.152: D4.C 46.74,15.62 46.74,12.95 T1.3 | SJ7.2 47.14,21.25 v47.14,20.95
N$10
  Top 0.152: SV1.3 27.63,54.61 28.75,53.49 29.67,53.49 32.8,56.62 37.53,56.62 37.57,56.58 38.31,56.58 38.35,56.62 44.41,56.62 44.59,56.43 46.27,56.43 48.26,58.42 CAN1.9
N$11
  Top 0.152: CON2.4 IC1.11 | R23.2 43.95,55.09 42.94,54.08 37.57,54.08 30.33,46.84 30.33,40.81 29.67,40.16 20.8,40.16 SV2.8
  Bottom 0.152: IC1.11 22.23,17.14 20.47,18.9 20.47,32.86 20.8,33.19 20.8,40.16 SV2.8
N$12
  Top 0.152: CON2.5 IC1.12
  Bottom 0.152: IC1.12 22.86,19.68 20.95,21.59 20.95,31.6 23.01,33.66 23.01,42.39 21.59,43.81 SV2.6 18.26,45.24 18.26,53.08 17.4,53.95 16.38,53.95 R22.2
N$13  (via drill 0.35)
  Top 0.152: v36.83,50.16 41.91,50.16 K5.10 45.8,48.97 45.8,50.66 47.62,52.49 R15.2
  Bottom 0.152: v36.83,50.16 SJ5.1
N$14  (via drill 0.35)
  Top 0.152: CON2.6 IC1.13 | v25.4,46.99 20.32,46.99 SV2.4
  Bottom 0.152: SV2.4 21.59,46.35 22.86,45.09 22.86,42.98 23.32,42.52 23.32,33.53 21.26,31.47 21.26,23.82 22.86,22.23 IC1.13 | R21.2 25.72,46.99 v25.4,46.99
N$15
  Bottom 0.152: SJ4.1 41.76,39.67 41.76,43.01 40.64,44.13 K4.10 40.95,45.09 43.33,47.47 43.33,48.09 45.41,50.16 R11.2
N$16
  Top 0.305: 2.1 70.65,2.54 71.89,3.79 74.03,3.79 75.27,2.54 CON9.2
  Bottom 0.305: CON9.2 IC5.2 SV6.3
N$17
  Bottom 0.152: 46.35,45.09 46.35,46.35 R14.2 | K3.10 46.35,45.09 | SJ3.1 43.18,40.96 44.3,42.08 44.3,43.03 46.35,45.09
N$18
  Bottom 0.305: SV6.1 IC5.1 | IC5.1 1.1 | IC5.1 CON9.1
N$19
  Bottom 0.152: K2.2 51.98,43.73 51.98,44.25 52.22,44.5 52.22,45.67 51.84,46.05 51.84,56.29 DJ1.2
N$20  (via drill 0.35)
  Top 0.152: Q1.D 41.91,29.84 | 41.91,29.84 36.83,29.84 D5.A 32.7,30.8 28.48,30.8 28.19,31.09 27.69,31.09 27.4,30.8 v26.67,30.8 | K1.2 41.91,29.84
  Bottom 0.152: v26.67,30.8 24.09,28.22 R16.2
N$21
  Bottom 0.152: K3.2 46.05,45.41 46.05,47.74 47.13,48.82 48.12,48.82 48.97,49.67 48.97,53.05 47.2,54.82 47.04,54.82 45.58,56.28 43.41,56.28 DJ2.2
N$22  (via drill 0.35)
  Top 0.152: R10.1 33.34,22.86 33.83,22.38 34.75,22.38 35.41,23.03 35.41,23.98 v36.83,25.4 42.55,25.4 K1.10 46.38,21.56 47.41,21.56 47.79,21.18 D8.C
  Bottom 0.152: SJ1.1 v36.83,25.4
N$23
  Top 0.152: CON1.6 IC1.6
  Bottom 0.152: IC1.6 17.78,13.34 17.78,15.44 17.88,15.55 17.88,25.82 17.78,25.93 17.78,31.9 18.26,32.38 18.26,34.12 17.14,35.24 SV2.11
N$24  (via drill 0.35)
  Top 0.152: v53.34,43.81 54.61,45.09 K2.10
  Bottom 0.152: SJ2.1 52.7,43.18 v53.34,43.81 53.34,46.04 54.46,47.16 54.46,48.09 53.34,49.21 R12.2
N$25
  Top 0.152: K6.2 3.81,51.44 Q3.D
  Bottom 0.152: Q3.D 12.7,53.34 D7.A | R20.2 2.54,50.63 K6.2
N$26  (via drill 0.35)
  Top 0.152: K4.2 39.06,39.04 47.12,39.04 47.42,38.73 v50.8,38.73
  Bottom 0.152: Q2.D 50.8,31.11 50.8,33.34 49.68,34.46 49.68,35.39 52.4,38.11 52.4,38.73 | K4.2 35.56,43.5 36.68,44.62 36.68,46.35 41.91,51.59 K5.2 DJ2.1 | v50.8,38.73 52.4,38.73 | 52.4,47.62 52.4,49.42 52.15,49.67 52.15,53.98 53.34,55.17 | D6.A 52.4,47.62 | 52.4,38.73 52.4,44.24 52.53,44.37 52.53,45.8 52.4,45.93 52.4,47.62 | 53.34,55.17 DJ1.1 | R18.2 53.42,55.17 53.34,55.17
N$27
  Top 0.152: CON1.5 IC1.5
  Bottom 0.152: SV2.9 15.88,37.47 15.88,27.4 17.58,25.7 17.58,15.67 IC1.5
N$28
  Top 0.152: R1.2 20.1,3.81 18.91,5 15.8,5 13.97,3.17 J1.2
N$29
  Bottom 0.305: CON10.1 IC5.5 | IC5.5 SV6.8 | IC5.5 5.1
N$30
  Top 0.152: CON1.3 IC1.3
  Bottom 0.152: IC1.3 15.44,20.75 15.44,42.11 SV2.5
N$31
  Top 0.305: 6.1 82.89,15.24 81.65,13.99 79.51,13.99 78.27,15.24 CON10.2
  Bottom 0.305: SV6.6 IC5.6 CON10.2
N$32
  Top 0.305: 7.1 70.42,15.24 71.69,13.97 74.23,13.97 CON10.3
  Bottom 0.305: CON10.3 IC5.7 SV6.4
N$33
  Top 0.152: S2.2 S2.1
  Bottom 0.152: S2.2 45.72,7.26 R3.2
N$34
  Top 0.152: R4.2 5.18,9.58 5.18,13.23 LED1.A 5.18,13.39 5.18,15.98 LED2.K 7.62,21.01 5.18,23.44 LED3.A
  Bottom 0.152: LED5.K 7.62,30.3 6.25,28.93 6.25,24.66 LED3.A
N$35
  Bottom 0.406: SV4.14 IC4.8 CON8.1 B8.1
N$36
  Top 0.152: LED7.K 27.99,27.23 R16.1
N$37
  Top 0.152: R18.1 55.58,54.94 55.58,55.88 55.58,55.91 55.58,57.28 56.55,58.26 LED8.K
N$38
  Bottom 0.152: R20.1 5.11,55.75 LED9.K
N$39
  Bottom 0.152: SJ7.1 47.17,23.5 C1.1
N$40
  Bottom 0.406: B9.1 81.85,57.78 CON8.2 IC4.9 SV4.12
N$41
  Bottom 0.406: B10.1 79.31,59.05 CON8.3 IC4.10 SV4.10
N$42
  Top 0.152: LED3.K 7.62,26.04 LED4.A 5.18,28.63 5.18,33.66 LED5.A
  Bottom 0.152: LED6.K 7.62,36.09 5.18,33.66 LED5.A | R5.2 5.18,5.77 5.18,7.9 6.4,9.12 6.4,10.49 8.84,12.93 8.84,22.23 7.62,23.44 LED3.K
N$43
  Bottom 0.406: B11.1 CON8.4 IC4.11 SV4.8
N$44
  Top 0.152: LED4.K 7.62,31.98 6.25,33.35 6.25,37.62 5.18,38.68 LED6.A | R6.2 5.18,2.59 5.18,4.09 6.4,5.31 6.4,12.01 7.62,13.23 LED1.K
  Bottom 0.152: LED1.K 7.62,15.98 5.18,18.41 | LED4.K 7.62,25.12 6.25,23.75 6.25,19.48 5.18,18.41 | 5.18,18.41 LED2.A
N$45
  Top 0.406: SV1.6 28.57,52.07 27.28,53.37 26.15,53.37 25.43,54.09 25.43,55.91 SV1.1
  Bottom 0.406: SJ8.1 26.48,57.15 SV1.1
N$46
  Bottom 0.406: B12.1 74.23,59.05 CON8.5 IC4.12 SV4.6
N$47
  Bottom 0.406: B13.1 71.69,57.78 CON8.6 IC4.13 SV4.4
N$48
  Top 0.152: CON3.3 IC2.3
  Bottom 0.152: SV3.5 26.67,35.24 27.79,34.12 27.79,31.82 27.33,31.37 27.33,28.22 27.84,27.71 27.84,17.14 30.38,14.61 CON3.3
N$49
  Bottom 0.406: B14.1 CON8.7 IC4.14 SV4.2
N$50
  Bottom 0.406: SV4.13 IC4.7 CON5.7 B7.1
N$51
  Bottom 0.406: B6.1 81.85,42.55 CON5.6 IC4.6 SV4.11
N$52
  Bottom 0.406: SV4.9 IC4.5 CON5.5 79.31,41.27 B5.1
N$53
  Bottom 0.406: B4.1 CON5.4 IC4.4 SV4.7
N$54
  Bottom 0.406: SV4.5 IC4.3 CON5.3 74.23,41.27 B3.1
N$55
  Bottom 0.406: B2.1 71.69,42.55 CON5.2 IC4.2 SV4.3
N$56
  Bottom 0.406: B1.1 CON5.1 IC4.1 SV4.1
N$57
  Bottom 0.305: CON10.4 IC5.8 | IC5.8 SV6.2 | 8.1 IC5.8
N$58
  Top 0.152: 80.53,23.53 IC3.8 | 80.53,21.09 CON7.4 | 80.53,22.55 85.04,22.55 86.56,21.03 88.24,21.03 E8.1
  Top 0.406: 80.53,21.09 80.53,22.55 80.53,23.53 | IC3.8 80.58,26.66 79.8,27.44 70.42,27.44 SV5.1
N$59
  Top 0.152: 72.91,31.3 IC3.4 | 72.91,33.74 CON6.4 73,33.83 74.37,35.2 85.04,35.2 86.56,33.68 88.24,33.68 E4.1
  Top 0.406: 72.91,33.74 72.91,31.3 | SV5.2 70.42,29.98 71.69,29.98 IC3.4
N$60
  Top 0.152: 78.09,23.53 IC3.7 | 78.09,21.09 CON7.3 78.18,21.03 79.4,19.81 81.08,19.81 82.14,20.88 84.43,20.88 E7.1
  Top 0.406: 78.09,21.09 78.09,23.53 | IC3.7 79.31,24.9 SV5.9
N$61
  Top 0.152: E6.1 69.34,20.88 70.87,20.88 71.93,19.81 74.22,19.81 75.44,21.03 CON7.2
  Top 0.406: CON7.2 IC3.6 74.23,24.9 SV5.5
N$62
  Top 0.152: 72.91,23.53 IC3.5 | 72.91,21.09 CON7.1 | E5.1 65.53,21.03 67.06,21.03 70.56,24.54 71.63,24.54 71.77,24.67
  Top 0.406: 72.91,21.09 72.91,23.53 71.77,24.67 71.69,24.75 SV5.3
N$63
  Top 0.152: 80.53,31.3 IC3.1 | 80.53,33.74 CON6.1 80.62,33.68 84.43,33.68 E3.1
  Top 0.406: 80.53,33.74 80.53,31.3 | IC3.1 79.31,29.98 78.04,29.98 SV5.8
N$64
  Top 0.152: 78.09,31.3 IC3.2 | 78.09,33.74 CON6.2
  Top 0.406: 78.09,33.74 78.09,31.3 | SV5.6 75.5,29.98 76.77,29.98 IC3.2
  Bottom 0.152: E2.1 69.34,33.53 69.34,33.22 73.76,28.8 74.22,28.8 SV5.6
N$65
  Top 0.406: CON6.3 IC3.3 74.23,29.98 72.96,29.98 SV5.4
  Bottom 0.152: E1.1 65.53,33.53 66.9,33.53 71.63,28.8 SV5.4
N$66
  Top 0.152: SV7.7 49.25,73.11 50.32,73.11 51.38,74.18 52.45,74.18 52.76,73.88 53.52,73.88 53.82,74.18 54.74,74.18 55.65,73.27 55.65,72.05 56.11,71.59 57.33,71.59 60.53,68.39 60.53,67.93 IC6.10
  Bottom 0.406: IC6.10 CON12.10
N$67
  Top 0.152: S1.2 28.57,6.71 | 28.57,6.71 S1.1 | 28.57,6.71 28.22,6.35 R2.2
N$68
  Top 0.152: SV7.3 54.28,72.96 54.28,72.05 53.06,70.83 53.06,67.93 IC6.7
  Bottom 0.406: CON12.7 IC6.7
N$69
  Bottom 0.152: SV7.2 56.72,70.37 55.96,70.37 54.89,69.3 53.67,69.3 53.52,69.46 52.45,69.46 50.62,67.63 IC6.6
  Bottom 0.406: CON12.6 IC6.6
N$70
  Bottom 0.152: SV7.1 56.72,72.96 55.96,72.96 54.59,71.59 51.23,71.59 50.47,70.83 50.47,70.07 48.49,68.08 48.03,68.08 IC6.5
  Bottom 0.406: CON12.5 IC6.5
N$71
  Bottom 0.406: CON12.3 IC6.3 42.88,69.16 SV7.12
N$72
  Bottom 0.406: CON12.2 IC6.2 40.34,69.16 SV7.14
N$73
  Bottom 0.406: CON12.1 IC6.1 37.8,69.16 SV7.13
N$74
  Bottom 0.406: CON12.4 IC6.4
N$75
  Bottom 0.406: CON12.8 IC6.8
N$76
  Bottom 0.406: CON12.9 IC6.9
N$77
  Bottom 0.406: IC6.11 CON11.1
N$78
  Bottom 0.406: CON11.2 IC6.12
N$79
  Bottom 0.406: CON11.3 IC6.13
N$80
  Bottom 0.406: IC6.14 CON11.4
N$81
  Bottom 0.406: CON11.5 IC6.15
N$82
  Bottom 0.406: IC6.16 CON11.6
N$83
  Bottom 0.406: CON11.7 IC6.17
N$84
  Bottom 0.406: IC6.18 CON11.8
N$85
  Bottom 0.406: CON11.9 IC6.19
N$86
  Bottom 0.406: IC6.20 CON11.10
N$87
  Bottom 0.152: SV8.3 14.48,71.63 18.9,71.63 19.66,70.87 19.66,70.1 21.79,67.97 IC7.9
N$88
  Top 0.152: IC7.8 19.2,67.97 17.07,70.1 17.07,75.25 IC7.22
  Bottom 0.152: SV8.2 10.82,73 11.73,73 12.95,71.78 13.72,71.78 14.63,72.69 14.63,73.46 16.61,75.44 IC7.22
N$89
  Top 0.152: 11.58,70.41 10.82,70.41 SV8.1 11.58,70.41 | 11.58,70.41 12.8,71.63 13.87,71.63 14.48,71.02 14.48,70.1 16.61,67.97 IC7.7
N$90
  Bottom 0.152: IC7.1 1.52,67.82 2.13,67.82 3.66,66.29 17.07,66.29 18.29,67.51 18.29,70.41 SV8.7
N$91
  Top 0.152: IC7.17 29.41,75.44 29.41,73.91 26.06,70.56 SV8.13
N$92
  Top 0.152: IC7.18 26.82,75.44 26.82,73.91 26.06,73.15 SV8.14
N$93
  Top 0.152: 65.84,74.07 64.77,75.13 L1.K | 65.84,74.07 65.99,73.91 65.99,68.43 SV9.2 | 65.84,74.07 69.49,77.72 L2.A
  Bottom 0.152: 83.82,73 86.26,70.56 88.54,70.56 L4.K | 83.82,73 81.38,70.56 79.1,70.56 L11.K 78.94,70.56 76.81,70.56 74.37,73 L12.A 74.22,73.15 69.65,77.72 L2.A | 83.82,73 L3.A
N$94
  Top 0.152: SV8.12 24.23,73.76 24.23,75.44 IC7.19
N$95
  Top 0.152: L7.K 81.53,77.72 83.82,77.72 L9.A | L2.K 69.65,75.29 71.78,75.29 74.22,77.72 L8.A
  Bottom 0.152: 68.43,74.07 69.49,75.13 L2.K | 68.43,74.07 64.92,70.56 64.92,67.97 65.99,66.9 65.99,66.45 SV9.1 | 68.43,74.07 64.77,77.72 L1.A | L7.K 78.94,75.29 76.81,75.29 74.37,77.72 L8.A | L10.K 88.54,75.29 86.26,75.29 83.82,77.72 L9.A
N$96
  pour Bottom: 1.27,78.74 34.29,78.74 34.29,64.77 1.27,64.77
N$97
  Top 0.152: 86.56,75.13 85.04,75.13 | 85.04,75.13 83.82,75.13 L9.K | 86.56,75.13 88.54,73.15 L4.A | 86.56,75.13 88.54,77.11 88.54,77.72 L10.A | 85.04,75.13 85.04,71.78 83.82,70.56 L3.K
  Bottom 0.152: 81.84,68.43 68.12,68.43 SV9.4 | 81.84,68.43 83.82,70.41 L3.K | 81.84,68.43 83.82,66.45 | 83.82,66.45 85.5,68.12 88.54,68.12 L5.A | 83.82,66.45 L6.K
N$98
  Top 0.152: SV9.3 68.12,66.45 70.26,66.45 L12.K 74.37,70.56 74.37,71.48 75.44,72.54 75.44,75.13 | L5.K 88.54,65.84 86.11,65.84 83.82,68.12 L6.A 83.82,68.28 79.1,73 L11.A 78.94,73.15 76.96,75.13 | 76.96,75.13 75.44,75.13 | 75.44,75.13 74.37,75.13 L8.K | 76.96,75.13 78.94,77.11 78.94,77.72 L7.A
N$99
  pour Bottom: 36.83,78.74 60.96,78.74 60.96,64.77 36.83,64.77
N$100
  pour Bottom: 63.5,78.74 90.17,78.74 90.17,64.77 63.5,64.77
N$101
  pour Bottom: 63.5,62.23 90.17,62.23 90.17,38.1 63.5,38.1
N$102
  pour Bottom: 63.5,35.56 90.17,35.56 90.17,19.05 63.5,19.05
N$103
  pour Bottom: 63.5,16.51 90.17,16.51 90.17,1.27 63.5,1.27
N$104
  pour Top: 63.5,16.51 90.17,16.51 90.17,1.27 63.5,1.27
N$105
  pour Top: 63.5,19.05 90.17,19.05 90.17,35.56 63.5,35.56
N$106
  pour Top: 63.5,62.23 90.17,62.23 90.17,38.1 63.5,38.1
N$107
  pour Top: 63.5,78.74 90.17,78.74 90.17,64.77 63.5,64.77
N$108
  Bottom 0.152: Q4.D 34.29,57.94 R21.1
N$109
  Bottom 0.152: Q5.D 30.33,59.85 28.09,57.61 28.09,56.03 27.94,55.88 21.59,55.88 19.68,57.78 15.08,57.78 R22.1
N$110
  Bottom 0.152: Q6.D 46.83,55.88 R23.1
P1
  Top 0.152: C4.1 52.07,10.79 55.88,10.79 | U1.D2 57.15,10.79 55.88,10.79 | C2.1 55.88,10.79
P2
  Top 0.152: U1.D3 57.46,14.61 56.34,13.49 55.42,13.49 54.3,14.61 C3.1
PRG_R
  Top 0.152: R17.1 54.19,23.5 55.39,22.3 56.37,22.3 57.07,23 57.07,23.42 U1.D7
  Bottom 0.152: R17.1 53.98,24.13 Q2.G 58.24,32.84 58.86,32.84 59.49,33.47 59.49,39.43 59.38,39.54 59.38,40.55 59.79,40.96 59.79,42.1 58.99,42.9 57.54,42.9 57.3,43.13 57.3,52.97 56.52,53.76 56.52,56.26 53.82,58.95 52.86,58.95 51.69,57.78 Q6.G 46.62,57.78 45.45,58.95 41.43,58.95 40.1,57.63 40.1,55.19 39.58,54.67 38.84,54.67 38.32,55.19 38.32,57.09 Q4.G Q5.G
PWR_EX
  Top 0.152: K6.1 6.04,52.7 7.16,53.82 8.08,53.82 9.2,52.7 15.24,52.7 17.14,50.8 SV2.1 18.1,48.9 19.22,50.01 21.71,50.01 24.13,47.6 25.65,47.6 26.67,46.58 26.67,43.81 SV3.2
PWR_R  (via drill 0.35)
  Top 0.152: v14.3,30.18 14.94,29.54 33.68,29.54 33.83,29.69 35.13,29.69 37.97,26.85 41.53,26.85 43.61,24.77 56.52,24.77 58.42,26.67 U1.D8
  Bottom 0.152: v14.3,30.18 13.97,30.51 13.97,42.01 12.06,43.92 R19.1 12.7,46.99 Q3.G
PWR_TY
  Top 0.152: CON1.1 IC1.1 20.42,20.85 39.47,20.85 IC2.8 CON4.4 | K6.5 K6.6
  Bottom 0.152: SJ6.2 5.08,43.81 6.35,42.55 K6.6 8.65,42.55 9.72,43.61 11.51,43.61 12.64,42.48 12.64,30.98 13.97,29.65 CON1.1
PWR_U  (via drill 0.35)
  Top 0.152: U1.D9 56.82,29.77 53.91,29.77 53.02,28.88 50.48,28.88 49.9,29.46 48.53,29.46 46.22,27.15 38.1,27.15 35.26,30 33.7,30 33.55,29.85 16.51,29.85 15.24,31.11 v13.36,31.11
  Bottom 0.152: v13.36,31.11 13.36,42.19 11.56,43.99 9.98,43.99 8.44,45.53 SJ6.1 5.08,51.44 6.35,52.7 K6.10
RST_EX  (via drill 0.35)
  Top 0.152: K1.1 44.45,27.46 38.79,27.46 35.76,30.48 v27.94,30.48 | SV2.7 18.1,41.27 19.22,42.39 20.15,42.39 21.27,41.27 SV3.1
  Bottom 0.152: SV3.1 28.09,39.85 28.09,30.63 v27.94,30.48
RST_R
  Top 0.152: Q1.G 52.07,28.57 53.34,27.3 54.61,27.3 R13.1
  Bottom 0.152: R13.1 57.15,27.3 57.15,23.5 U1.D6
RST_TY
  Top 0.152: CON1.4 IC1.4 22.62,17.14 23.79,18.31 27.84,18.31 29.21,19.68 CON3.1 IC2.1
  Bottom 0.152: K1.5 34.48,28.39 SJ1.2 34.48,23.68 K1.6 33.02,22.23 IC2.1

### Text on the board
Top: +5V | Top
Bottom: GND | Bot
tPlace: ATTiny88 | by Hardi | by Hardi | + | by Hardi | + | 1 | Charliplexing / LED Test | + | + | 1 | + | + | 1 | 1 | 1 | by Hardi | Read | + | Prog. | + | Error | + | + | + | Servo Debug | Heart / Beat | + | by Hardi | Normal / Reset / Funkt. | + | Reset / as / IO Pin | by Hardi | Tiny UniProg | 30.10.19 | by Hardi | Restart Tiny | Chg Reset Pin
tNames: Pwr Rel. | Data Rel. | Data Rel.
bNames: CAN +5V | by Hardi | Close SJ1 - SJ6 / if used without / Relais | V 1.1 | Tiny UniProg | Opt. C

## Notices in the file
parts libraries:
SparkFun-Connectors: Licensing: Creative Commons ShareAlike 4.0 International - https://creativecommons.org/licenses/by-sa/4.0
